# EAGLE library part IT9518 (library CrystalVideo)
ITE IT9518 MFQN 64 pin package COFDM SOC modulator
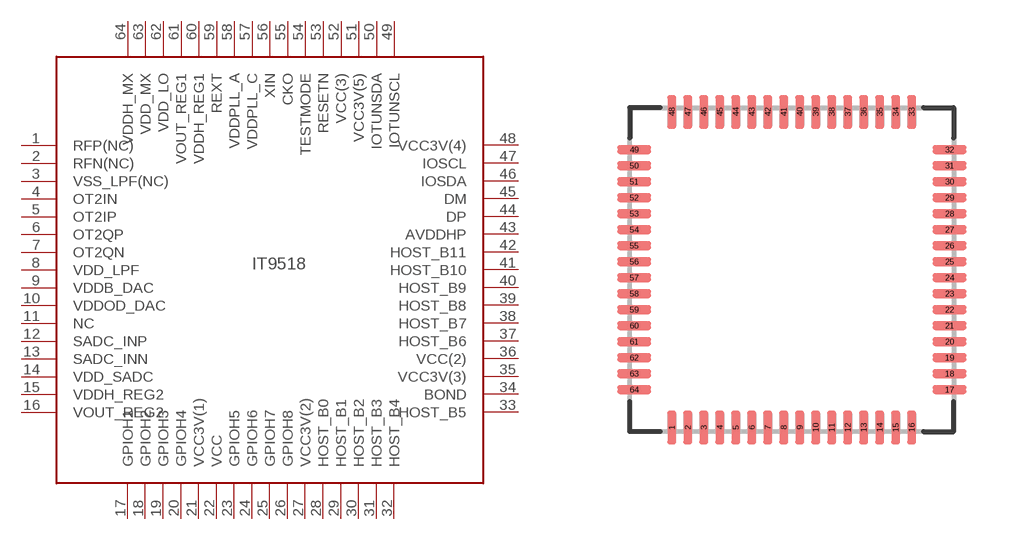
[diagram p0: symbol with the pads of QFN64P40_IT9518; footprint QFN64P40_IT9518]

Designator prefix -

## IT9518  [QFN64P40_IT9518]
1  RFP(NC)
2  RFN(NC)
3  VSS_LPF(NC)
4  OT2IN
5  OT2IP
6  OT2QP
7  OT2QN
8  VDD_LPF
9  VDDB_DAC
10  VDDOD_DAC
11  NC
12  SADC_INP
13  SADC_INN
14  VDD_SADC
15  VDDH_REG2
16  VOUT_REG2
17  GPIOH1
18  GPIOH2
19  GPIOH3
20  GPIOH4
21  VCC3V(1)
22  VCC
23  GPIOH5
24  GPIOH6
25  GPIOH7
26  GPIOH8
27  VCC3V(2)
28  HOST_B0
29  HOST_B1
30  HOST_B2
31  HOST_B3
32  HOST_B4
33  HOST_B5
34  BOND
35  VCC3V(3)
36  VCC(2)
37  HOST_B6
38  HOST_B7
39  HOST_B8
40  HOST_B9
41  HOST_B10
42  HOST_B11
43  AVDDHP
44  DP
45  DM
46  IOSDA
47  IOSCL
48  VCC3V(4)
49  IOTUNSCL
50  IOTUNSDA
51  VCC3V(5)
52  VCC(3)
53  RESETN
54  TESTMODE
55  CKO
56  XIN
57  VDDPLL_C
58  VDDPLL_A
59  REXT
60  VDDH_REG1
61  VOUT_REG1
62  VDD_LO
63  VDD_MX
64  VDDH_MX

## Footprint QFN64P40_IT9518 (pad centres in mm)
ITE IT9518 Quad Flat No-Lead (QFN), 0.40 mm pitch; square, 16 pin X 16 pin, 8.00 mm L X 8.00 mm W X 0.80 mm H
smd 0.22 x 0.84: 1 -3,-3.945; 2 -2.6,-3.945; 3 -2.2,-3.945; 4 -1.8,-3.945; 5 -1.4,-3.945; 6 -1,-3.945; 7 -0.6,-3.945; 8 -0.2,-3.945; 9 0.2,-3.945; 10 0.6,-3.945; 11 1,-3.945; 12 1.4,-3.945; 13 1.8,-3.945; 14 2.2,-3.945; 15 2.6,-3.945; 16 3,-3.945; 33 3,3.945; 34 2.6,3.945; 35 2.2,3.945; 36 1.8,3.945; 37 1.4,3.945; 38 1,3.945; 39 0.6,3.945; 40 0.2,3.945; 41 -0.2,3.945; 42 -0.6,3.945; 43 -1,3.945; 44 -1.4,3.945; 45 -1.8,3.945; 46 -2.2,3.945; 47 -2.6,3.945; 48 -3,3.945
smd 0.84 x 0.22: 17 3.945,-3; 18 3.945,-2.6; 19 3.945,-2.2; 20 3.945,-1.8; 21 3.945,-1.4; 22 3.945,-1; 23 3.945,-0.6; 24 3.945,-0.2; 25 3.945,0.2; 26 3.945,0.6; 27 3.945,1; 28 3.945,1.4; 29 3.945,1.8; 30 3.945,2.2; 31 3.945,2.6; 32 3.945,3; 49 -3.945,3; 50 -3.945,2.6; 51 -3.945,2.2; 52 -3.945,1.8; 53 -3.945,1.4; 54 -3.945,1; 55 -3.945,0.6; 56 -3.945,0.2; 57 -3.945,-0.2; 58 -3.945,-0.6; 59 -3.945,-1; 60 -3.945,-1.4; 61 -3.945,-1.8; 62 -3.945,-2.2; 63 -3.945,-2.6; 64 -3.945,-3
